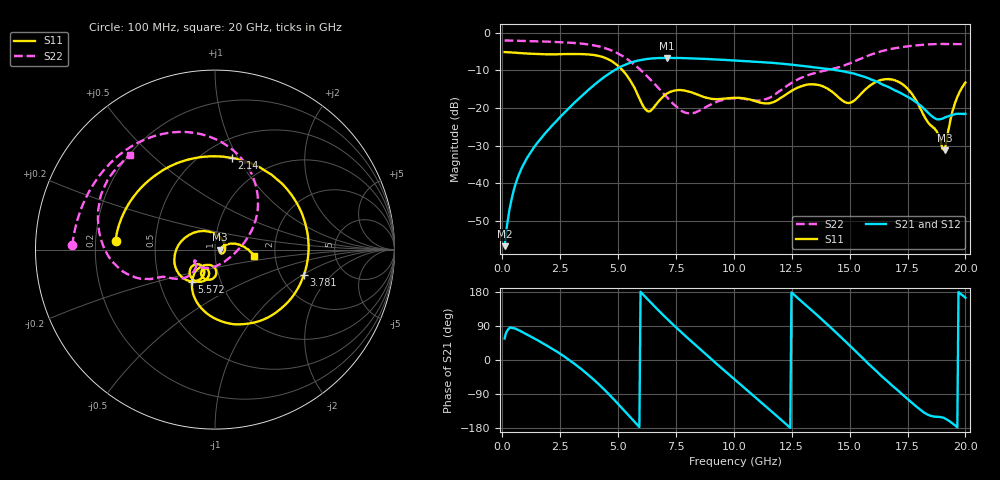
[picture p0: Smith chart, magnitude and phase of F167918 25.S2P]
!  2-Port S-parameters saved by WinCal
! VAR MeasName=S-Parameters (CALIBRATED_DATA) read from VNA (N5242A)
! VAR MeasDate=2016-11-22 10:25:58
! VAR NAME=F167918 25
! VAR FILENAME=F167918 25.S2P
! VAR DATE=2016-11-22 10:25:58
! VAR PHYS_PORTS=1,2
# Hz S DB R 50
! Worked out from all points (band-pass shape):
!   401 points, 100 MHz to 20 GHz, reference 50 ohm
!   highest |S21| = -6.63 dB at 7.115 GHz (marker M1); lowest = -56.8 dB at 100 MHz (marker M2)
!   |S21| within 3 dB of the highest: 4.922 GHz to 14.12 GHz (9.194 GHz wide, 96.6 % of centre)
!   lowest |S11| = -31.2 dB at 19.1 GHz (marker M3), VSWR 1.06, Z = 52.8 - j0.1 ohm
!   |S11| at or under -10 dB: 5.204 GHz to end of sweep
!   |S22| runs from -21.4 to -2.0 dB; largest |S21 - S12| = 0.004
!   S11 on the Smith chart (normalised r, x): 100 MHz: 0.29, +0.04; 2.14 GHz: 0.67, +0.94; 3.781 GHz: 2.66, -1.04; 5.572 GHz: 0.73, -0.28; 20 GHz: 1.55, -0.11
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1e8  -5.09 175.2  -56.78 56.8  -56.29 55.3  -2.00 178.3
7.4675e8  -5.35 145.5  -37.30 77.6  -37.22 77.1  -2.11 168.1
2.13975e9  -5.69 79.7  -24.76 30.1  -24.74 29.8  -2.35 145.7
3.43325e9  -5.64 5.8  -16.75 -25.0  -16.76 -25.0  -2.84 119.7
3.7815e9  -5.77 -16.2  -14.84 -42.8  -14.83 -42.7  -3.12 111.1
4.62725e9  -7.17 -71.8  -10.75 -91.8  -10.72 -91.8  -4.44 86.5
5.5725e9  -13.14 -125.3  -7.84 -153.7  -7.83 -153.9  -7.78 55.3
6.269e9  -20.78 -111.2  -6.92 160.8  -6.91 160.6  -11.64 33.1
6.7665e9  -18.12 -86.7  -6.68 129.5  -6.68 129.5  -14.84 17.1
7.11475e9  -16.13 -91.8  -6.63 108.7  -6.64 108.8  -17.15 4.1
7.91075e9  -15.40 -112.9  -6.72 63.2  -6.69 63.2  -21.21 -43.4
8.657e9  -16.96 -121.9  -6.88 22.1  -6.87 22.1  -20.24 -96.1
1.005e10  -17.26 -119.8  -7.35 -52.1  -7.34 -52.1  -17.39 -146.1
1.09455e10  -18.23 -122.7  -7.68 -99.1  -7.66 -99.2  -17.97 -149.7
1.19405e10  -17.65 -105.0  -8.13 -152.2  -8.10 -152.3  -15.62 -134.6
1.338325e10  -13.69 -124.9  -9.07 129.8  -9.04 130.1  -10.88 -145.8
1.517425e10  -18.12 -119.8  -10.80 28.0  -10.80 28.2  -7.69 -156.7
1.67165e10  -12.34 -153.2  -14.49 -60.8  -14.48 -60.7  -4.37 -178.4
1.7612e10  -15.61 150.2  -17.39 -108.4  -17.29 -108.6  -3.50 166.7
1.91045e10  -31.21 -2.0  -22.59 -153.9  -22.48 -153.6  -2.95 143.3
1.955225e10  -18.60 16.4  -21.66 -172.5  -21.53 -172.5  -2.98 137.4
2e10  -13.21 -8.8  -21.54 164.2  -21.41 164.8  -2.99 131.8
